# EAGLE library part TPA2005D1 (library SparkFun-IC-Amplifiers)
1.4W MONO CLASS-D AUDIO POWER AMPLIFIER The TPA2005D1 is a 1.4-W high efficiency filter-free class-D audio power amplifier in a BGA, QFN, or MSOP package that requires only three external components. Datasheet: http://focus.ti.com/lit/ds/symlink/tpa2005d1.pdf 1.4 W Into 8 ? From a 5V Supply at THD = 10% (Typ) Maximum Battery Life and Minimum Heat Efficiency With an 8-? Speaker: 84% at 400 mW, 79% at 100 mW 2.8-mA Quiescent Current 0.5-mA Shutdown Current Ideal for Wireless or Cellular Handsets and PDAs Capable of Driving an 8-? Speaker (2.5 V ? VDD ? 5.5 V) and a 4-? Speaker (2.5 V ? VDD ? 4.2 V) Only Three External Components Optimized PWM Output Stage Eliminates LC Output Filter Internally Generated 250-kHz Switching Frequency Eliminates Capacitor and Resistor Improved PSRR (-71 dB at 217 Hz) and Wide Supply Voltage (2.5 V to 5.5 V) Eliminates Need for a Voltage Regulator Fully Differential Design Reduces RF Rectification and Eliminates Bypass Capacitor Improved CMRR Eliminates Two Input Coupling Capacitors SparkFun Products SparkFun Mono Audio Amp Breakout - TPA2005D1 (BOB-11044) Note: SparkFun currenly only uses the QFN style part
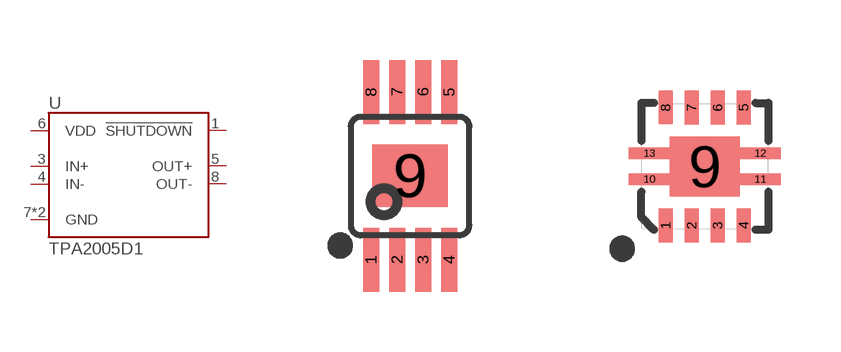
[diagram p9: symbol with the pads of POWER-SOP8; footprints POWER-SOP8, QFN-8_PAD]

Designator prefix U

## TPA2005D1DGN (PROD_ID: NA-XXXXX; VALUE: TPA2005D1)  [POWER-SOP8]
1  !SHUTDOWN  in
3  IN+
4  IN-
5  OUT+
6  VDD  pwr
7  GND  pwr
8  OUT-
9  GND  pwr

## TPA2005D1DRB (PROD_ID: IC-10975; VALUE: TPA2005D1)  [QFN-8_PAD]
1  !SHUTDOWN  in
3  IN+
4  IN-
5  OUT+
6  VDD  pwr
7  GND  pwr
8  OUT-
9  GND  pwr
10  GND  pwr
11  GND  pwr
12  GND  pwr
13  GND  pwr

## Footprint POWER-SOP8 (pad centres in mm)
8M, 8-Lead, 0.118" Wide, Miniature Small Outline Package MSOP 8M-Package doc1097.pdf
smd 0.4 x 1.6: 1 -0.975,-2.1; 2 -0.325,-2.1; 3 0.325,-2.1; 4 0.975,-2.1; 5 0.975,2.1; 6 0.325,2.1; 7 -0.325,2.1; 8 -0.975,2.1
smd 1.89 x 1.57: 9 0,0

## Footprint QFN-8_PAD (pad centres in mm)
smd 0.35 x 0.85: 1 -0.975,-1.475; 2 -0.325,-1.475; 3 0.325,-1.475; 4 0.975,-1.475; 5 0.975,1.475; 6 0.325,1.475; 7 -0.325,1.475; 8 -0.975,1.475
smd 1.75 x 1.5: 9 0,0
smd 1.025 x 0.28: 10 -1.387,-0.325; 11 1.387,-0.325; 12 1.387,0.325; 13 -1.387,0.325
